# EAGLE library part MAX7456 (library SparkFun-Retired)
Monochrome NTSC/PAL on-screen display generator (SPI)
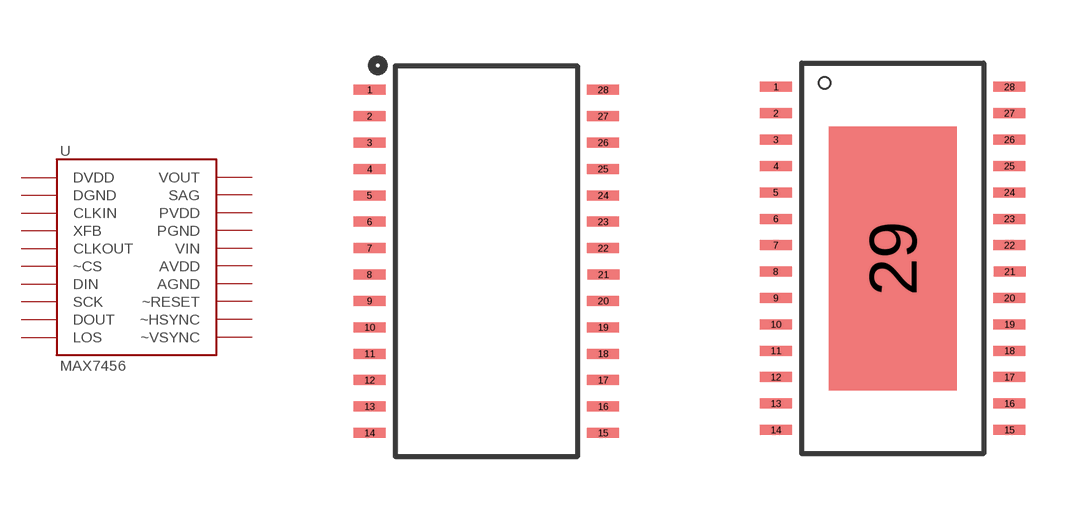
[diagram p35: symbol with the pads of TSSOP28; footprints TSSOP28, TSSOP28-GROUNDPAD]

Designator prefix -

## MAX7456  [TSSOP28]
3  DVDD
4  DGND
5  CLKIN
6  XFB
7  CLKOUT
8  ~CS
9  DIN
10  SCK
11  DOUT
12  LOS
17  ~VSYNC
18  ~HSYNC
19  ~RESET
20  AGND
21  AVDD
22  VIN
23  PGND
24  PVDD
25  SAG
26  VOUT

## MAX7456GROUNDPAD  [TSSOP28-GROUNDPAD]
Pads as for TSSOP28

## Footprint TSSOP28 (pad centres in mm)
smd 0.8 x 0.25: 1 -2.921,4.623; 2 -2.921,3.962; 3 -2.921,3.302; 4 -2.921,2.642; 5 -2.921,1.981; 6 -2.921,1.321; 7 -2.921,0.66; 8 -2.927,0; 9 -2.921,-0.66; 10 -2.921,-1.321; 11 -2.921,-1.981; 12 -2.921,-2.642; 13 -2.921,-3.302; 14 -2.921,-3.962; 15 2.921,-3.962; 16 2.921,-3.302; 17 2.921,-2.642; 18 2.921,-1.981; 19 2.921,-1.321; 20 2.921,-0.66; 21 2.927,0; 22 2.921,0.66; 23 2.921,1.321; 24 2.921,1.981; 25 2.921,2.642; 26 2.921,3.302; 27 2.921,3.962; 28 2.921,4.623

## Footprint TSSOP28-GROUNDPAD (pad centres in mm)
smd 0.8 x 0.25: 1 -2.921,4.298; 2 -2.921,3.637; 3 -2.921,2.977; 4 -2.921,2.317; 5 -2.921,1.656; 6 -2.921,0.996; 7 -2.921,0.335; 8 -2.927,-0.325; 9 -2.921,-0.985; 10 -2.921,-1.646; 11 -2.921,-2.306; 12 -2.921,-2.967; 13 -2.921,-3.627; 14 -2.921,-4.287; 15 2.921,-4.287; 16 2.921,-3.627; 17 2.921,-2.967; 18 2.921,-2.306; 19 2.921,-1.646; 20 2.921,-0.985; 21 2.927,-0.325; 22 2.921,0.335; 23 2.921,0.996; 24 2.921,1.656; 25 2.921,2.317; 26 2.921,2.977; 27 2.921,3.637; 28 2.921,4.298
smd 3.2 x 6.6: 29 0,0.005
